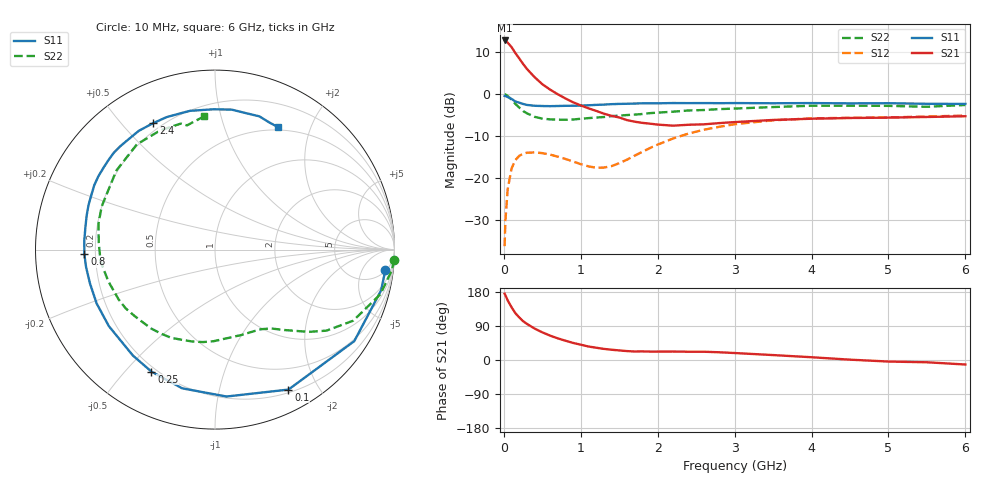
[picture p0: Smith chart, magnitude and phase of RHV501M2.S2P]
! SIEMENS Small Signal Semiconductors
! BFR106
! Si NPN RF Bipolar Junction Transistor in SOT23
! VCE = 0.5 V  IC = 1.2 mA
! Common Emitter S-Parameters:  August  1996
# GHz  S  MA  R  50
!  f  S11  S21  S12  S22
! GHz  MAG  ANG  MAG  ANG  MAG  ANG  MAG  ANG
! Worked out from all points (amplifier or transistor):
!   36 points, 10 MHz to 6 GHz, reference 50 ohm
!   highest |S21| = 12.8 dB at 10 MHz (marker M1)
!   |S21| within 3 dB of that: start of sweep to 149.8 MHz
!   unconditionally stable (mu >= 1): 795.6 MHz to end of sweep
!   at 250 MHz: K = 0.32, MSG = 10.7 dB, |S12| = -14.2 dB
!   at 1.4 GHz: K = 1.57, MAG = 1.6 dB, |S12| = -17.2 dB
!   at 6 GHz: K = 1.02, MAG = -1.0 dB, |S12| = -5.1 dB
!   S11 on the Smith chart (normalised r, x): 10 MHz: 6, -15; 100 MHz: 0.23, -1.63; 250 MHz: 0.18, -0.59; 800 MHz: 0.16, -0.02; 2.4 GHz: 0.17, +0.61; 6 GHz: 0.46, +1.53
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0.01  0.956 -6.8  4.389 174.9  0.0154 87.0  0.9974 -3.2
0.02  0.9529 -13.8  4.339 171.1  0.0308 81.7  0.9939 -6.3
0.05  0.9286 -33.3  4.127 157.4  0.0736 70.1  0.9547 -15.1
0.1  0.8807 -62.3  3.661 139.3  0.13 54.5  0.8661 -27.2
0.15  0.8211 -85.5  3.105 123.5  0.1641 41.5  0.7681 -36.0
0.2  0.7942 -103.3  2.68 112.4  0.1842 32.9  0.6947 -41.3
0.25  0.7666 -117.5  2.304 102.5  0.1953 26.0  0.632 -45.7
0.3  0.7467 -127.8  2.007 95.3  0.2006 21.2  0.593 -49.1
0.4  0.7291 -144.2  1.6 83.0  0.2025 13.8  0.5382 -54.7
0.5  0.7245 -155.6  1.32 73.0  0.1986 8.9  0.5124 -60.0
0.6  0.7217 -165.0  1.139 64.4  0.1908 5.7  0.5019 -65.9
0.8  0.7283 -178.0  0.893 50.9  0.1693 4.1  0.4966 -78.3
1.1  0.7397 165.2  0.68 35.6  0.1381 12.6  0.5197 -97.5
1.3  0.753 156.2  0.587 29.3  0.1334 26.3  0.5356 -110.3
1.6  0.7705 143.9  0.492 23.5  0.1657 44.9  0.5653 -128.8
2.2  0.7863 122.7  0.422 22.3  0.2968 48.1  0.62 -163.4
2.4  0.7843 116.0  0.433 21.8  0.3399 44.7  0.6412 -174.2
2.8  0.7832 105.0  0.453 20.4  0.4095 36.1  0.6652 167.3
3.5  0.7818 90.6  0.494 13.0  0.4893 21.4  0.7042 141.3
4.5  0.7795 76.7  0.521 0.9  0.5245 4.5  0.7308 114.8
5.5  0.77 66.7  0.536 -6.0  0.5436 -4.5  0.7095 102.7
6  0.7673 63.0  0.547 -11.9  0.5571 -11.0  0.7455 94.6
